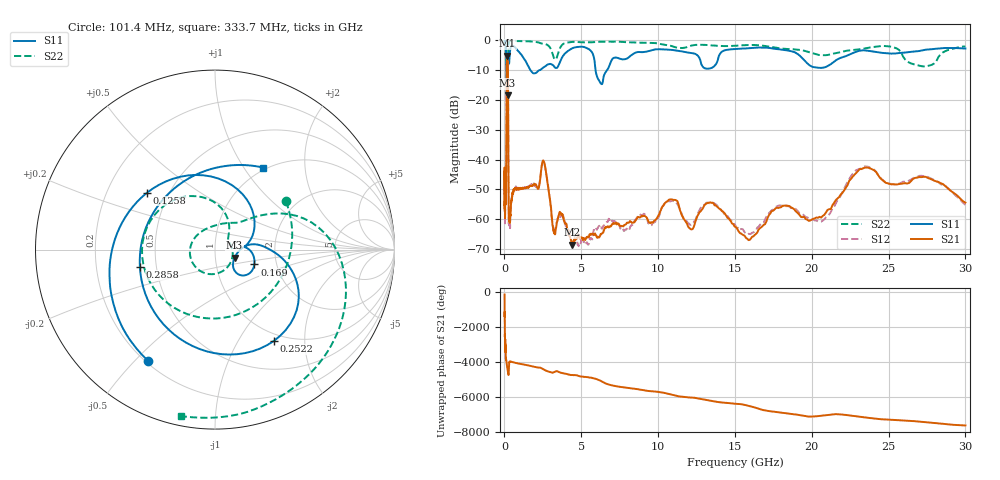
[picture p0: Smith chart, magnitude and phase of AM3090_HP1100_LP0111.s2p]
! Date/Time: Thu, Feb 28, 2019 2:06 PM
! Network Analyzer: Agilent Technologies E8364B Rev: A.07.50.67
! Sweep from 0.010 to 30.000 GHz, 1601 Points, Sweep Type: LOG
! Power Supply: 5.022 V, 0.002 A
# Hz S DB R 50
!freq MagS11 AngS11 MagS21 AngS21 MagS12 AngS12 MagS22 AngS22
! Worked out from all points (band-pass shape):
!   1601 points, 10 MHz to 30 GHz, reference 50 ohm
!   highest |S21| = -5.26 dB at 176.8 MHz (marker M1); lowest = -68.5 dB at 4.391 GHz (marker M2)
!   |S21| within 3 dB of the highest: 142 MHz to 221.5 MHz (79.5 MHz wide, 43.7 % of centre)
!   lowest |S11| = -18.6 dB at 203.4 MHz (marker M3), VSWR 1.27, Z = 62 - j5.62 ohm
!   |S11| at or under -10 dB: 136.3 MHz to 227 MHz (90.7 MHz wide, 49.9 % of centre); 1.676 GHz to 2.35 GHz (673.8 MHz wide, 33.5 % of centre); 5.926 GHz to 6.696 GHz (770.6 MHz wide, 12.2 % of centre)
!   |S22| runs from -21.0 to -0.2 dB; largest |S21 - S12| = 0.012
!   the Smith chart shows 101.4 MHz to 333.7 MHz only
!   S11 on the Smith chart (normalised r, x): 101.4 MHz: 0.21, -0.54; 125.8 MHz: 0.38, +0.32; 169 MHz: 1.53, -0.27; 252.2 MHz: 0.89, -1.43; 285.8 MHz: 0.40, -0.10; 333.7 MHz: 0.96, +1.22
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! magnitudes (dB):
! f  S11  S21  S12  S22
! 10 MHz  -0.3  -44.0  -44.8  -0.6
! 38.04 MHz  -0.4  -58.7  -60.9  -1.4
! 47.65 MHz  -0.6  -49.5  -47.9  -1.5
! 101.4 MHz  -2.8  -53.2  -53.1  -6.4
! 125.8 MHz  -6.1  -24.7  -24.7  -7.8
! 144.7 MHz  -14.8  -7.3  -7.3  -18.1
! 169 MHz  -12.6  -5.3  -5.3  -18.2
! 176.8 MHz  -12.5  -5.3  -5.2  -17.0
! 203.4 MHz  -18.6  -6.0  -5.9  -18.0
! 229.3 MHz  -9.4  -11.2  -11.1  -11.8
! 252.2 MHz  -4.4  -35.2  -35.4  -2.7
! 285.8 MHz  -7.3  -59.7  -61.1  -1.0
! 333.7 MHz  -5.5  -59.9  -60.5  -0.5
! 550.5 MHz  -2.0  -51.2  -51.3  -0.3
! 2.084 GHz  -10.9  -48.8  -49.1  -0.7
! 2.571 GHz  -9.1  -40.7  -40.9  -1.3
! 3.204 GHz  -8.7  -63.6  -64.4  -5.8
! 4.391 GHz  -2.9  -68.5  -64.0  -0.7
! 7.926 GHz  -6.3  -61.6  -63.5  -0.8
! 15.97 GHz  -2.8  -66.8  -64.9  -1.7
! 23.48 GHz  -3.5  -42.7  -42.3  -2.8
! 30 GHz  -2.9  -54.4  -55.2  -2.2
